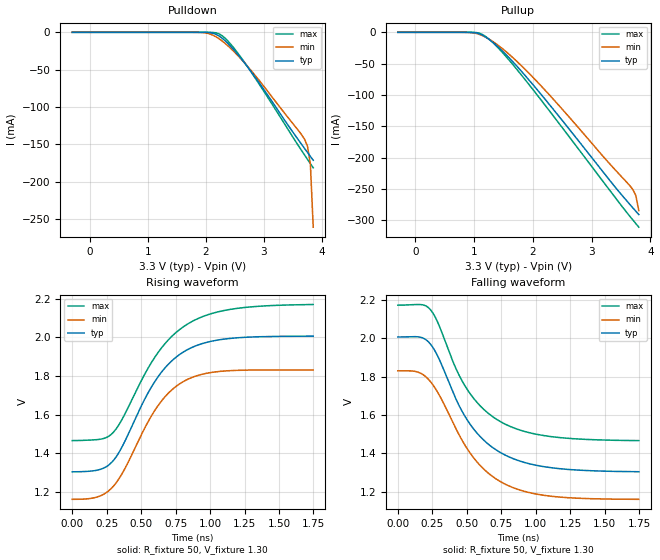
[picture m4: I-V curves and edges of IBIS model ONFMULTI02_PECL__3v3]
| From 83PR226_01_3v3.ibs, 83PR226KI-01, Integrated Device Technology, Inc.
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[Model] ONFMULTI02_PECL__3v3
Model_type   Output_ECL
Polarity   Non-Inverting
|   typ   min   max
C_comp   2pF   1.5pF   2.5pF
Vmeas = 1.60V
Rref = 50
Cref = 0
Vref = 1.3V
|   typ   min   max
[Voltage range]   3.3V   3.135V   3.465V
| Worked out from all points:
|   rising waveform, R_fixture 50, V_fixture 1.30: 20-80 % time 334ps typ, 316ps min, 375ps max; typ from 1.3 V to 2.01 V
|   falling waveform, R_fixture 50, V_fixture 1.30: 20-80 % time 346ps typ, 354ps min, 339ps max; typ from 2.01 V to 1.3 V
[Pulldown]
|Voltage   I (typ)   I (min)   I (max)
|Note, modeling breaks down at 250mA and above.  This is well beyond the functional   |
|operating range of the device.  Should this scenario occur, catastrophic failure and   |
|possible damage to the device and/or board is of higher concern than the I-V curve   |
|behavior.  The IBIS checker will flag currents in excess of 10A with warnings.  Lines   |
|with currents in excess of 0.35 A have been commented out.  The points still remain|
|available to the user if the user desires to use them.   |
|-2.70000e+00   5.90688e+00   4.78743e+00   7.17557e+00
|-2.10000e+00   3.98431e+00   3.34390e+00   4.72258e+00
|-1.50000e+00   2.06424e+00   1.90300e+00   2.27172e+00
|-9.00000e-01   1.51425e-01   4.67372e-01   5.24346e-03
-300mV    30.93nA    4.722uA    119.8pA
1.929V    -10.54uA   -227.9uA   -152.7nA
2.126V    -1.19mA    -3.898mA   -187.5uA
2.225V    -4.65mA    -8.342mA   -1.859mA
2.323V    -10.56mA   -14.13mA   -7.175mA
2.521V    -26.68mA   -28.47mA   -24.59mA
2.767V    -51.16mA   -49.84mA   -51.44mA
3.606V    -145.2mA   -132.5mA   -153.1mA
3.704V    -155.8mA   -143.4mA   -164.7mA
3.753V    -161.1mA   -152.8mA   -170.4mA
3.803V    -166.3mA   -176.6mA   -176mA
3.852V    -171.5mA   -261.2mA   -181.6mA
| 3.90138e+00   -1.76732e-01   -4.44584e-01   -1.87123e-01
| 3.95069e+00   -1.82005e-01   -6.29962e-01   -1.92613e-01
| 4.00000e+00   -1.87428e-01   -8.15337e-01   -1.98078e-01
| 4.01000e+00   -1.88587e-01   -8.52930e-01   -1.99185e-01
| 4.52800e+00   -2.13399e+00   -2.80117e+00   -1.06737e+00
| 5.04600e+00   -4.72362e+00   -4.74981e+00   -4.36727e+00
| 5.56400e+00   -7.31841e+00   -6.70087e+00   -7.67562e+00
| 6.08200e+00   -9.92709e+00   -8.65887e+00   -1.10059e+01
| 6.60000e+00   -1.25638e+01   -1.06309e+01   -1.43799e+01
[Pullup]
|Voltage   I (typ)   I (min)   I (max)
|Note, modeling breaks down at 250mA and above.  This is well beyond the functional   |
|operating range of the device.  Should this scenario occur, catastrophic failure and   |
|possible damage to the device and/or board is of higher concern than the I-V curve   |
|behavior.  The IBIS checker will flag currents in excess of 10A with warnings.  Lines   |
|with currents in excess of 0.35 A have been commented out.  The points still remain|
|available to the user if the user desires to use them.   |
|-2.70000e+00   5.90688e+00   4.78743e+00   7.17557e+00
|-2.10000e+00   3.98431e+00   3.34390e+00   4.72258e+00
|-1.50000e+00   2.06424e+00   1.90300e+00   2.27172e+00
|-9.00000e-01   1.51425e-01   4.67372e-01   5.24346e-03
-300mV    30.93nA    4.722uA    119.8pA
992.1mV   -419.8uA   -1.017mA   -107.3uA
1.091V    -2.5mA     -3.419mA   -1.423mA
1.239V    -10.22mA   -10.04mA   -9.694mA
1.387V    -21.45mA   -19.22mA   -22.61mA
1.584V    -39.49mA   -34.13mA   -43.06mA
2.028V    -86.45mA   -74.4mA    -94.51mA
3.359V    -242.1mA   -215.1mA   -258.3mA
3.655V    -275.1mA   -245.2mA   -294mA
3.704V    -280.4mA   -251.2mA   -299.7mA
3.753V    -285.6mA   -260.6mA   -305.3mA
3.803V    -290.8mA   -284.6mA   -310.9mA
| 3.85207e+00   -2.96015e-01   -3.69253e-01   -3.16380e-01
| 3.90138e+00   -3.01235e-01   -5.52734e-01   -3.21823e-01
| 3.95069e+00   -3.06489e-01   -7.38194e-01   -3.27224e-01
| 4.00000e+00   -3.11892e-01   -9.23648e-01   -3.32599e-01
| 4.01000e+00   -3.13046e-01   -9.61256e-01   -3.33688e-01
| 4.52800e+00   -2.25814e+00   -2.91033e+00   -1.20065e+00
| 5.04600e+00   -4.84648e+00   -4.85954e+00   -4.49743e+00
| 5.56400e+00   -7.43616e+00   -6.80976e+00   -7.79627e+00
| 6.08200e+00   -1.00300e+01   -8.76259e+00   -1.11020e+01
| 6.60000e+00   -1.26324e+01   -1.07202e+01   -1.44224e+01
[Ramp]
|   typ   min   max
dV/dt_r   0.421/0.334n   0.401/0.316n   0.422/0.375n
dV/dt_f   0.421/0.346n   0.401/0.354n   0.424/0.339n
R_load =   50.0000
[Rising Waveform]
R_fixture = 50
V_fixture = 1.30   | VCC_typ - 2V
V_fixture_max = 1.465   | VCC_max - 2V
V_fixture_min = 1.135   | VCC_min - 2V
C_fixture = 0.0p
| Time   typ   min   max
0s        1.304V     1.161V     1.465V
182.2ps   1.312V     1.173V     1.47V
294.3ps   1.359V     1.226V     1.505V
374.9ps   1.451V     1.31V      1.593V
600.9ps   1.773V     1.623V     1.898V
702.5ps   1.864V     1.714V     1.99V
816.3ps   1.928V     1.775V     2.059V
961.7ps   1.971V     1.812V     2.111V
1.146ns   1.994V     1.827V     2.144V
1.748ns   2.006V     1.83V      2.169V
[Falling Waveform]
R_fixture = 50
V_fixture = 1.30   | VCC_typ - 2V
V_fixture_max = 1.465   | VCC_max - 2V
V_fixture_min = 1.135   | VCC_min - 2V
C_fixture = 0.0p
| Time   typ   min   max
0s        2.006V     1.83V      2.171V
145.4ps   2.007V     1.823V     2.175V
234.7ps   1.971V     1.776V     2.15V
285.5ps   1.913V     1.723V     2.089V
413.4ps   1.697V     1.542V     1.856V
495.7ps   1.584V     1.433V     1.742V
611.4ps   1.478V     1.328V     1.638V
748ps     1.403V     1.252V     1.564V
1.091ns   1.328V     1.179V     1.49V
1.748ns   1.305V     1.162V     1.467V
